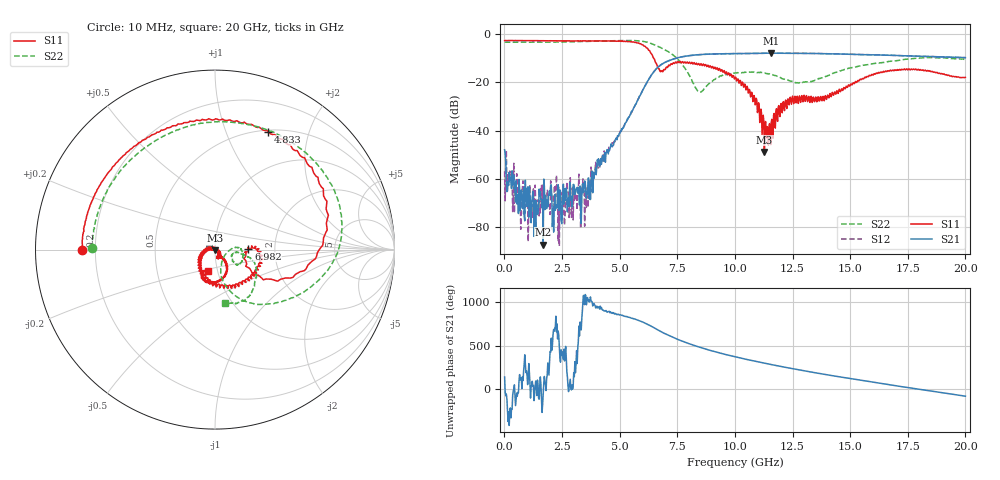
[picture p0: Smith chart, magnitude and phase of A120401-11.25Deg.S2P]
!  2-Port S-parameters saved by WinCal
! VAR MeasName=S-Parameters (CALIBRATED_DATA) read from VNA (N5244A)
! VAR MeasDate=11/21/2012 9:56:09 AM
! VAR NAME=A120401-11.25Deg
! VAR FILENAME=A120401-11.25Deg.S2P
! VAR DATE=11/21/2012 9:56:09 AM
! VAR PHYS_PORTS=1,2
# Hz S MA R 50
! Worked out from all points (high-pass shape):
!   801 points, 10 MHz to 20 GHz, reference 50 ohm
!   highest |S21| = -7.83 dB at 11.55 GHz (marker M1); lowest = -87.3 dB at 1.684 GHz (marker M2)
!   |S21| within 3 dB of the highest: 7.174 GHz to end of sweep
!   lowest |S11| = -48.9 dB at 11.28 GHz (marker M3), VSWR 1.01, Z = 50 - j0.357 ohm
!   |S11| at or under -10 dB: 6.485 GHz to end of sweep
!   |S22| runs from -24.0 to -2.6 dB; largest |S21 - S12| = 0.0048
!   S11 on the Smith chart (normalised r, x): 10 MHz: 0.15, -0.00; 4.833 GHz: 0.52, +1.42; 6.982 GHz: 1.46, +0.02; 20 GHz: 0.90, -0.22
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1e7  0.7385 -179.9  0.003992 142.0  0.00142 24.5  0.6849 179.4
1.849125e8  0.7413 176.4  0.000728 99.6  0.001045 -166.6  0.6853 175.5
7.846125e8  0.7388 164.8  0.0002397 140.4  0.0006807 -100.1  0.6849 161.1
1.684162e9  0.7329 147.1  4.312e-05 -51.4  0.0003059 -45.7  0.6865 139.5
2.183912e9  0.7322 136.8  0.0004714 -17.1  0.0007272 -137.4  0.6882 127.2
2.333838e9  0.7299 133.7  0.0007511 -49.6  5.028e-05 36.2  0.6886 123.5
3.358325e9  0.7251 109.9  0.0004092 93.4  0.0006721 -35.7  0.7068 97.7
4.832588e9  0.7206 65.6  0.006618 149.8  0.006474 144.5  0.7343 54.6
5.832088e9  0.6508 15.6  0.04822 72.1  0.04636 72.3  0.7298 16.7
6.681662e9  0.1948 -28.5  0.2116 -40.1  0.2119 -39.9  0.5544 -24.4
6.981512e9  0.1859 1.8  0.2619 -81.7  0.2622 -81.7  0.4717 -37.9
7.756125e9  0.2606 -19.7  0.3428 -170.1  0.3441 -170.3  0.222 -72.6
8.455775e9  0.2389 -50.4  0.3769 125.3  0.3754 125.3  0.06314 -36.5
1.0005e10  0.1197 -138.1  0.3966 14.2  0.3973 14.2  0.1572 -6.7
1.085458e10  0.04784 -173.5  0.3985 -35.6  0.3995 -35.7  0.1625 -25.3
1.127936e10  0.003599 -96.3  0.4029 -59.1  0.4019 -59.1  0.1564 -31.0
1.155422e10  0.005103 -114.2  0.4058 -74.0  0.4048 -73.9  0.1464 -35.1
1.230385e10  0.04549 -47.6  0.4018 -112.5  0.4032 -112.6  0.1123 -29.9
1.335332e10  0.03837 -63.4  0.4007 -163.2  0.4002 -163.3  0.1057 -8.9
1.515242e10  0.09838 -48.8  0.3819 116.6  0.3829 116.4  0.2061 -13.9
1.667666e10  0.1713 -79.6  0.3661 53.4  0.3668 53.2  0.2727 -32.0
2e10  0.1271 -107.6  0.3262 -79.0  0.3272 -79.2  0.2999 -79.8
